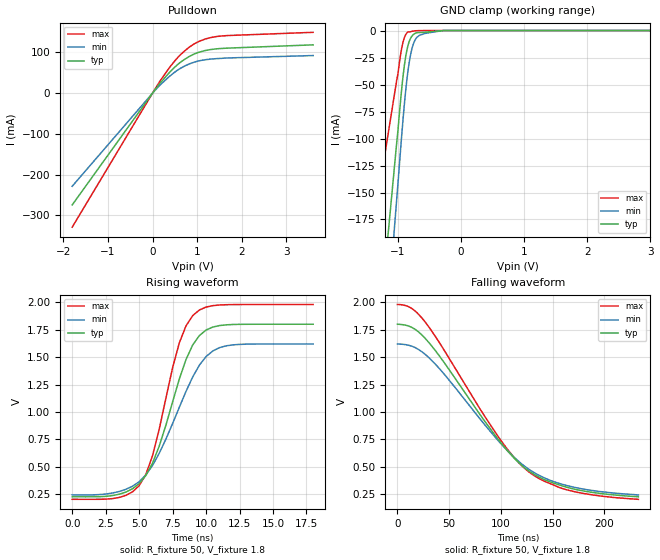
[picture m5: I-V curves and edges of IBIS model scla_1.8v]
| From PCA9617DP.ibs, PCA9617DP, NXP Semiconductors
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[Model]   scla_1.8v
Model_type Open_drain
Vref=1.800E+00
Rref=1.350E+03
Cref=5.000E-11
Vmeas=9.000E-01
C_comp   9.000E-13   8.790E-13   9.210E-13
[Voltage Range]   1.800E+00   1.620E+00   1.980E+00
[POWER Clamp Reference]   1.800E+00   1.620E+00   1.980E+00
[GND Clamp Reference]   0.000E+00   0.000E+00   0.000E+00
[Pullup Reference]   1.800E+00   1.620E+00   1.980E+00
[Pulldown Reference]   0.000E+00   0.000E+00   0.000E+00
[Temperature Range]   25   85   -40
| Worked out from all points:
|   slope of the pulldown table from 0 to 0.27 V, typ, clamps not added: 7.27 ohm
|   rising waveform, R_fixture 50, V_fixture 1.8: 20-80 % time 2.5ns typ, 3.09ns min, 2.11ns max; typ from 0.227 V to 1.8 V
|   falling waveform, R_fixture 50, V_fixture 1.8: 20-80 % time 74.4ns typ, 76ns min, 74.1ns max; typ from 1.8 V to 0.227 V
[GND Clamp]
-1.8V     -588.7mA   -735.2mA   -331.1mA
-1.02V    -103.6mA   -155.9mA   -45.9mA
-1V       -91.94mA   -141.4mA   -39.8mA
-960mV    -65.44mA   -111mA     -22.68mA
-920mV    -42.32mA   -82.04mA   -10.65mA
-880mV    -24.82mA   -56.73mA   -4.033mA
-840mV    -13.47mA   -36.58mA   -1.256mA
-780mV    -5.193mA   -17.02mA   -711.4uA
-740mV    -3.017mA   -10.04mA   -351.8uA
-700mV    -2.013mA   -6.247mA   -174.5uA
-280mV    0A         0A         0A
3.6V      0A         0A         0A
[Pulldown]
-1.8V     -274.1mA   -228.3mA   -328.7mA
140mV     20.39mA    16.66mA    24.94mA
480mV     61.94mA    50.04mA    76.7mA
600mV     73.62mA    59.26mA    91.49mA
740mV     84.49mA    67.63mA    105.6mA
900mV     94.37mA    74.85mA    118.6mA
1.04V     100.5mA    79.26mA    127mA
1.18V     104.6mA    82.01mA    132.8mA
1.44V     108.8mA    84.77mA    139.1mA
3.6V      118.6mA    92.34mA    149.3mA
[Rising Waveform]
R_fixture = 50
V_fixture = 1.8
V_fixture_min = 1.62
V_fixture_max = 1.98
0s        226.7mV    243.8mV    203.6mV
3.5ns     249.8mV    274.5mV    220.2mV
5ns       346.6mV    364.2mV    327.6mV
6ns       533.4mV    512.2mV    601mV
8ns       1.3V       1.042V     1.63V
8.5ns     1.478V     1.187V     1.785V
9.5ns     1.697V     1.427V     1.93V
10.5ns    1.774V     1.556V     1.97V
11.5ns    1.795V     1.603V     1.978V
18ns      1.8V       1.62V      1.98V
[Falling Waveform]
R_fixture = 50
V_fixture = 1.8
V_fixture_min = 1.62
V_fixture_max = 1.98
0s        1.8V       1.62V      1.98V
13ns      1.775V     1.602V     1.949V
26.5ns    1.675V     1.528V     1.825V
47ns      1.427V     1.325V     1.536V
97.5ns    750mV      738.5mV    775.1mV
113.5ns   573mV      581.6mV    577.3mV
126.5ns   466.2mV    481.6mV    458.2mV
141ns     388.3mV    404.1mV    373.6mV
164ns     313.3mV    328.7mV    289.8mV
233ns     226.7mV    243.8mV    203.6mV
[Ramp]
dV/dt_r   9.4399E-01/2.4940E-09   8.2569E-01/3.0750E-09   1.0658E+00/2.0920E-09
dV/dt_f   9.4399E-01/7.4320E-08   8.2569E-01/7.5937E-08   1.0658E+00/7.4117E-08
R_load = 50
